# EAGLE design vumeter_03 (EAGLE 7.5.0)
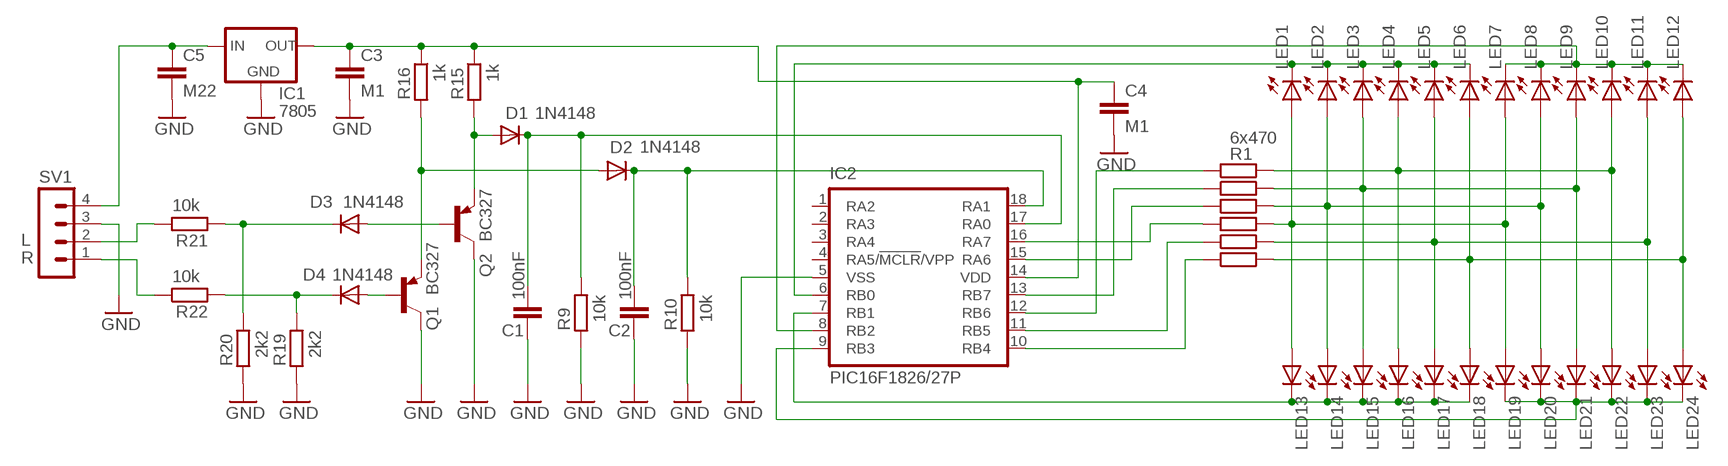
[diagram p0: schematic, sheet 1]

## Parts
C1  100nF  C-EU050-024X044  [C050-024X044]
C2  100nF  C-EU050-024X044  [C050-024X044]
C3  M1  C-EU050-024X044  [C050-024X044]
C4  M1  C-EU050-024X044  [C050-024X044]
C5  M22  C-EU050-024X044  [C050-024X044]
D1  1N4148  DIODE-D-7.5  [D-7.5]
D2  1N4148  DIODE-D-7.5  [D-7.5]
D3  1N4148  DIODE-D-7.5  [D-7.5]
D4  1N4148  DIODE-D-7.5  [D-7.5]
IC1  7805  78XXL  [78XXL]
IC2  PIC16F1826/27P  [DIL18]
LED1  LED5MM  [LED5MM]
LED2  LED5MM  [LED5MM]
LED3  LED5MM  [LED5MM]
LED4  LED5MM  [LED5MM]
LED5  LED5MM  [LED5MM]
LED6  LED5MM  [LED5MM]
LED7  LED5MM  [LED5MM]
LED8  LED5MM  [LED5MM]
LED9  LED5MM  [LED5MM]
LED10  LED5MM  [LED5MM]
LED11  LED5MM  [LED5MM]
LED12  LED5MM  [LED5MM]
LED13  LED5MM  [LED5MM]
LED14  LED5MM  [LED5MM]
LED15  LED5MM  [LED5MM]
LED16  LED5MM  [LED5MM]
LED17  LED5MM  [LED5MM]
LED18  LED5MM  [LED5MM]
LED19  LED5MM  [LED5MM]
LED20  LED5MM  [LED5MM]
LED21  LED5MM  [LED5MM]
LED22  LED5MM  [LED5MM]
LED23  LED5MM  [LED5MM]
LED24  LED5MM  [LED5MM]
Q1  BC327  [TO92-EBC]
Q2  BC327  [TO92-EBC]
R1  470  R-EU_0207/10  [0207/10]
R2  470  R-EU_0207/10  [0207/10]
R3  470  R-EU_0207/10  [0207/10]
R4  470  R-EU_0207/10  [0207/10]
R5  470  R-EU_0207/10  [0207/10]
R6  470  R-EU_0207/10  [0207/10]
R9  10k  R-EU_0207/10  [0207/10]
R10  10k  R-EU_0207/10  [0207/10]
R15  1k  R-EU_0207/10  [0207/10]
R16  1k  R-EU_0207/10  [0207/10]
R19  2k2  R-EU_0207/10  [0207/10]
R20  2k2  R-EU_0207/10  [0207/10]
R21  10k  R-EU_0207/10  [0207/10]
R22  10k  R-EU_0207/10  [0207/10]
SV1  MA04-1  [MA04-1]

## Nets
AN0: C1.1 D1.C IC2.17(RA0) R9.1
AN1: C2.1 D2.C IC2.18(RA1) R10.1
ANODY_L1: IC2.6(RB0) LED1.K(C) LED2.K(C) LED3.K(C) LED4.K(C) LED5.K(C) LED6.K(C)
ANODY_L2: IC2.8(RB2) LED7.K(C) LED8.K(C) LED9.K(C) LED10.K(C) LED11.K(C) LED12.K(C)
ANODY_R1: IC2.7(RB1) LED13.K(C) LED14.K(C) LED15.K(C) LED16.K(C) LED17.K(C) LED18.K(C)
ANODY_R2: IC2.9(RB3) LED19.K(C) LED20.K(C) LED21.K(C) LED22.K(C) LED23.K(C) LED24.K(C)
GND: C1.2 C2.2 C3.2 C4.2 C5.2 IC1.GND IC2.5(VSS) Q1.C Q2.C R9.2 R10.2 R19.2 R20.2 SV1.3
N$1: LED1.A LED7.A LED13.A LED19.A R4.2
N$2: LED2.A LED8.A LED14.A LED20.A R3.2
N$3: LED5.A LED11.A LED17.A LED23.A R5.2
N$4: LED4.A LED10.A LED16.A LED22.A R1.2
N$5: D4.A Q1.B
N$6: C5.1 IC1.IN SV1.4
N$7: D2.A Q1.E R16.2
N$8: LED6.A LED12.A LED18.A LED24.A R6.2
N$9: IC2.10(RB4) R6.1
N$10: IC2.11(RB5) R5.1
N$11: LED3.A LED9.A LED15.A LED21.A R2.2
N$12: IC2.16(RA7) R4.1
N$13: D1.A Q2.E R15.2
N$14: IC2.15(RA6) R3.1
N$15: IC2.13(RB7) R2.1
N$16: IC2.12(RB6) R1.1
N$17: D3.A Q2.B
N$18: R21.1 SV1.2
N$19: R22.1 SV1.1
N$20: C3.1 C4.1 IC1.OUT IC2.14(VDD) R15.1 R16.1
N$22: D3.C R20.1 R21.2
N$23: D4.C R19.1 R22.2
Unconnected: IC2.1(RA2) IC2.2(RA3) IC2.3(RA4) IC2.4(RA5/!MCLR!/VPP)

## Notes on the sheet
- 6x470
- L
- R

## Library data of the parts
C1-C5 = rcl:C-EU: CAPACITOR, European symbol
D1-D4 = diode:DIODE-: DIODE
IC1 = v-reg:78XXL: VOLTAGE REGULATOR
IC2 = microchip:PIC16*F1826/27: 18/20/28-Pin Flash Microcontrollers with nanoWatt XLP Technology Source: www.microchip.com PIC16F1827.pdf
LED1-LED24 = led:LED: LED
Q1 Q2 = transistor-pnp:BC327*: PNP Transistror
R1-R6 R9 R10 R15 R16 R19-R22 = rcl:R-EU_: RESISTOR, European symbol
SV1 = con-lstb:MA04-1: PIN HEADER

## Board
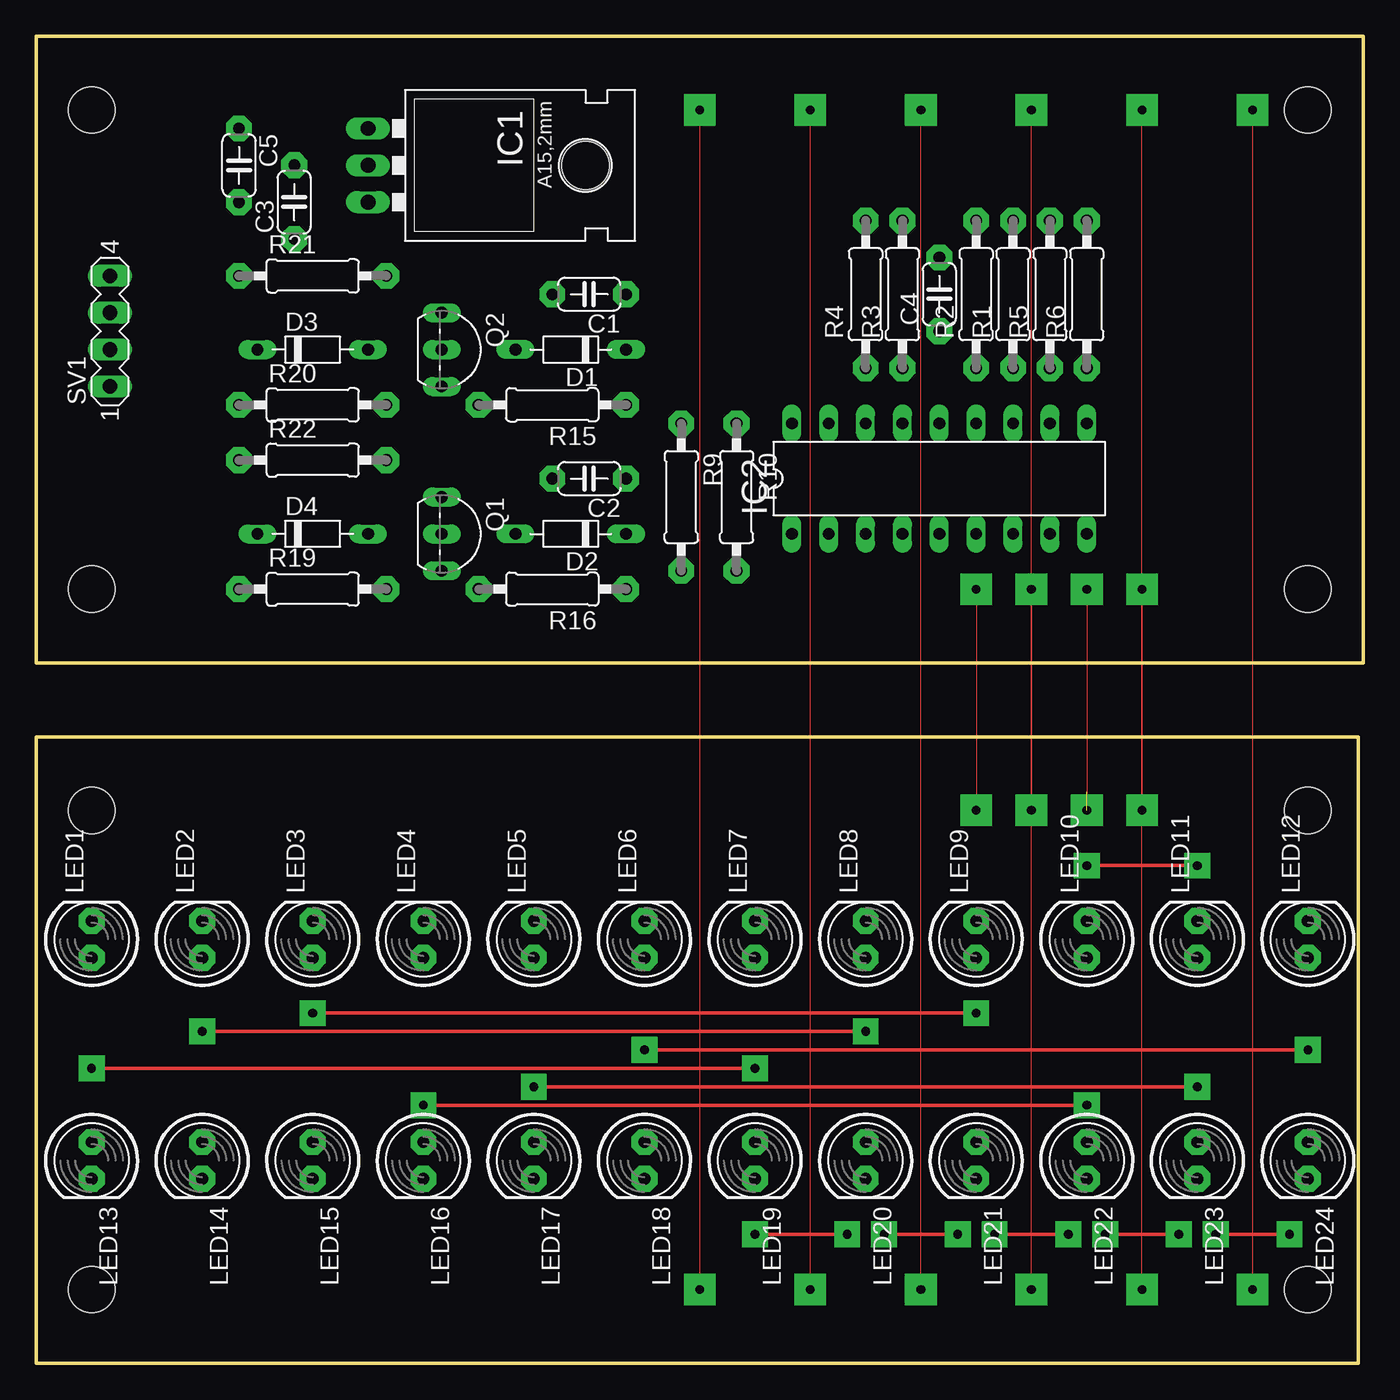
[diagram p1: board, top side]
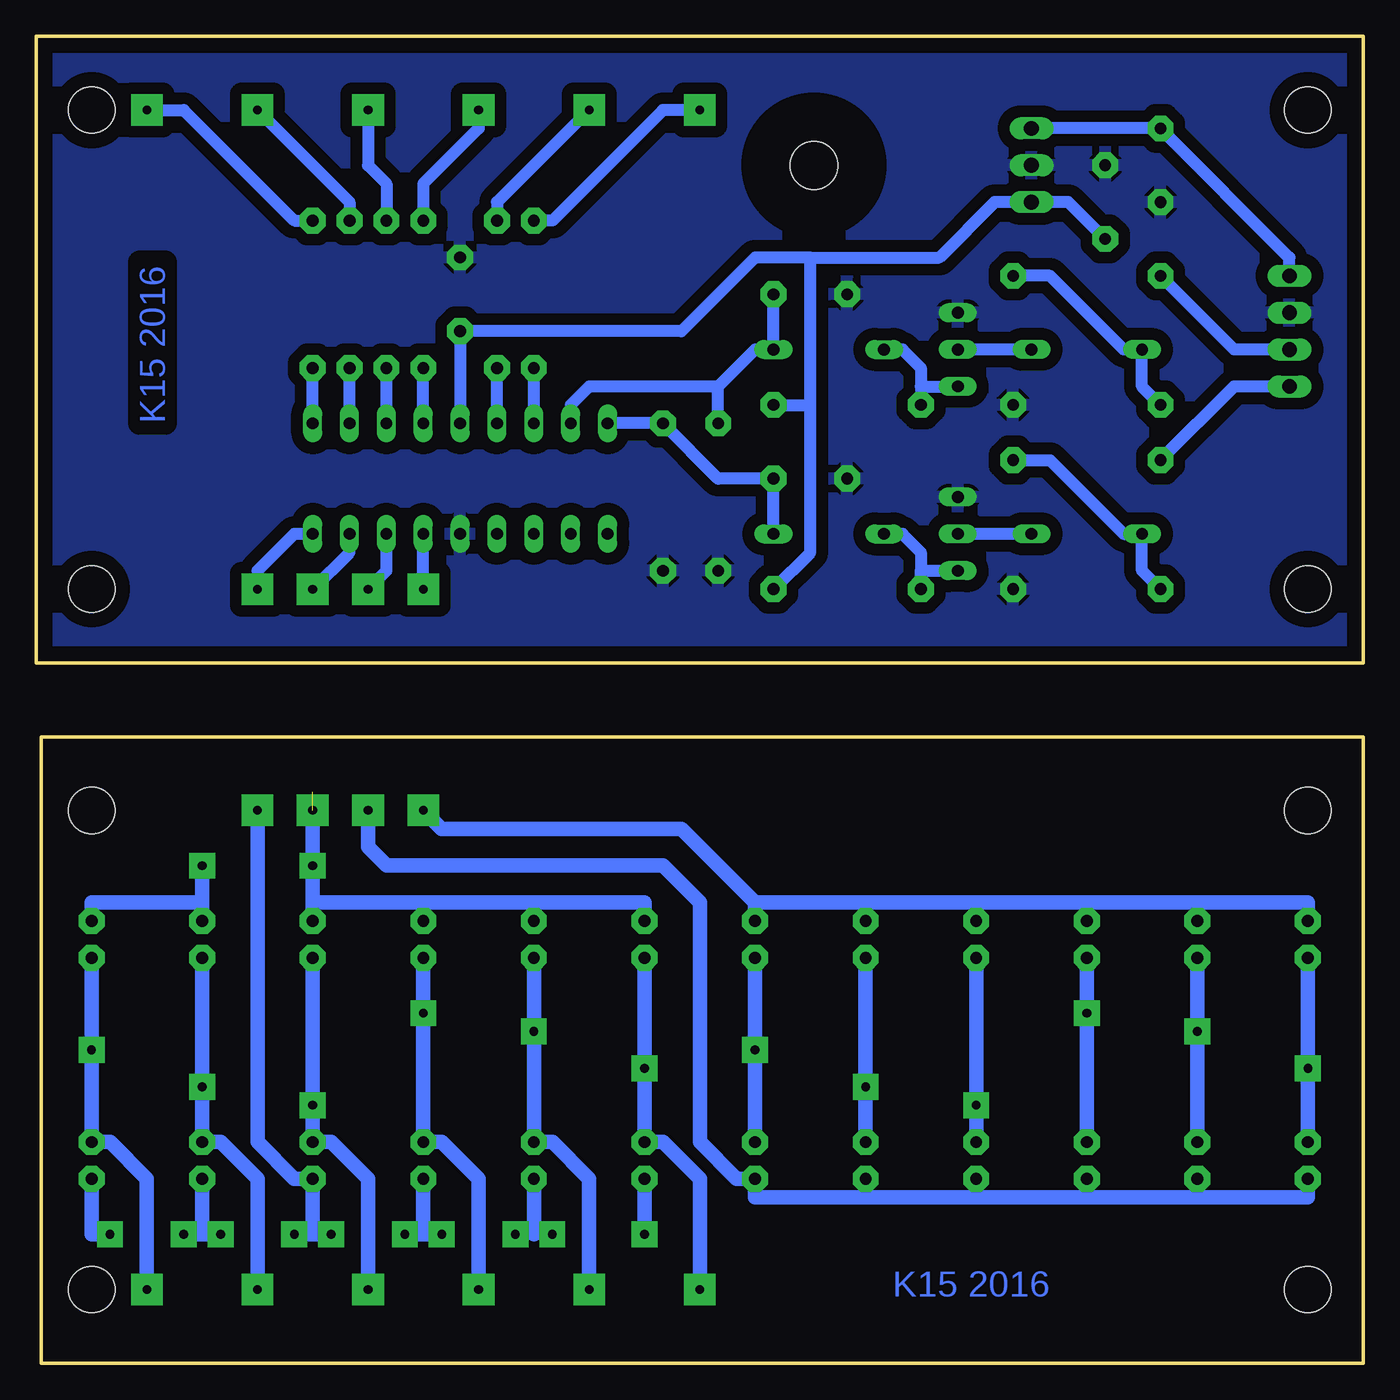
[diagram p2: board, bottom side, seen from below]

Size 91.44 x 91.44 mm. Coordinates in mm from the lower left corner, seen from the top.
Outline: 0,0 91.11,0 91.11,43.17 0,43.17 0,0
Outline: 0,48.26 91.44,48.26 91.44,91.44 0,91.44 0,48.26
Copper layers (1*16): Top 0.035mm / dielectric 1.5mm / Bottom 0.035mm
Design rules "default": minimum track width 10mil, minimum drill 24mil, track to track 8mil, track to pad 8mil, pad to pad 8mil, via to via 8mil, smd to smd 8mil, copper to edge 40mil, drill to drill 8mil, minimum pad ring 10mil, minimum via ring 8mil, stop-mask expansion 4mil, vias tented up to drill 0mil, thermal gap 10mil
Holes 3.2 mm at 3.81,38.1 87.63,5.08 87.63,53.34 3.81,53.34 87.63,38.1 3.81,5.08 87.63,86.36 3.81,86.36

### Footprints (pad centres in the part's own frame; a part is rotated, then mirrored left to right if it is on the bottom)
C050-024X044 = drill 0.813 pad 1.778 octagon: 1 -2.54,0; 2 2.54,0
D-7.5 = drill 0.813 long: A 3.81,0; C -3.81,0
78XXL = drill 1.016 long: GND 0,-3.81; IN -2.54,-3.81; OUT 2.54,-3.81 | hole 3.302: 0,11.176
DIL18 = drill 0.813 long: 1 -10.16,-3.81; 2 -7.62,-3.81; 3 -5.08,-3.81; 4 -2.54,-3.81; 5 0,-3.81; 6 2.54,-3.81; 7 5.08,-3.81; 8 7.62,-3.81; 9 10.16,-3.81; 10 10.16,3.81; 11 7.62,3.81; 12 5.08,3.81; 13 2.54,3.81; 14 0,3.81; 15 -2.54,3.81; 16 -5.08,3.81; 17 -7.62,3.81; 18 -10.16,3.81
LED5MM = drill 0.813 pad 1.778 octagon: A -1.27,0; K 1.27,0
TO92-EBC = drill 0.813 long: B 0,-1.27; C -2.54,-1.27; E 2.54,-1.27
0207/10 = drill 0.813 pad 1.778 octagon: 1 -5.08,0; 2 5.08,0
MA04-1 = drill 1.016 long: 1 -3.81,0; 2 -1.27,0; 3 1.27,0; 4 3.81,0

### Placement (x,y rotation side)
C1  38.1,73.66 180 top
C2  38.1,60.96 180 top
C3  17.78,80.01 90 top
C4  62.23,73.66 90 top
C5  13.97,82.55 270 top
D1  36.83,69.85 180 top
D2  36.83,57.15 180 top
D3  19.05,69.85 0 top
D4  19.05,57.15 0 top
IC1  26.67,82.55 270 top
IC2  62.23,60.96 0 top
LED1  3.81,29.21 90 top
LED2  11.43,29.21 90 top
LED3  19.05,29.21 90 top
LED4  26.67,29.21 90 top
LED5  34.29,29.21 90 top
LED6  41.91,29.21 90 top
LED7  49.53,29.21 90 top
LED8  57.15,29.21 90 top
LED9  64.77,29.21 90 top
LED10  72.39,29.21 90 top
LED11  80.01,29.21 90 top
LED12  87.63,29.21 90 top
LED13  3.81,13.97 270 top
LED14  11.43,13.97 270 top
LED15  19.05,13.97 270 top
LED16  26.67,13.97 270 top
LED17  34.29,13.97 270 top
LED18  41.91,13.97 270 top
LED19  49.53,13.97 270 top
LED20  57.15,13.97 270 top
LED21  64.77,13.97 270 top
LED22  72.39,13.97 270 top
LED23  80.01,13.97 270 top
LED24  87.63,13.97 270 top
Q1  29.21,57.15 270 top
Q2  29.21,69.85 270 top
R1  67.31,73.66 90 top
R2  64.77,73.66 90 top
R3  59.69,73.66 90 top
R4  57.15,73.66 90 top
R5  69.85,73.66 90 top
R6  72.39,73.66 90 top
R9  44.45,59.69 270 top
R10  48.26,59.69 270 top
R15  35.56,66.04 180 top
R16  35.56,53.34 180 top
R19  19.05,53.34 0 top
R20  19.05,66.04 0 top
R21  19.05,74.93 0 top
R22  19.05,62.23 0 top
SV1  5.08,71.12 90 top

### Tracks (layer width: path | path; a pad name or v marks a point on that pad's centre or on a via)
AN0
  Bottom 0.813: C1.1 D1.C 41.91,69.85 44.45,67.31 | IC2.17 54.61,66.04 53.34,67.31 44.45,67.31 | R9.1 44.45,67.31
AN1
  Bottom 0.813: D2.C C2.1 44.45,60.96 R10.1 IC2.18
ANODY_L1  (via drill 0.6 pad 2.18)
  Top 0: v64.77,53.34 v64.77,38.1
  Bottom 0.813: v64.77,53.34 IC2.6
  Bottom 1.016: 11.43,31.75 3.81,31.75 LED1.K | 11.43,31.75 19.05,31.75 | 19.05,31.75 26.67,31.75 | 26.67,31.75 34.29,31.75 | 34.29,31.75 41.91,31.75 | v64.77,38.1 63.5,36.83 46.99,36.83 41.91,31.75 | LED2.K 11.43,31.75 | LED3.K 19.05,31.75 | LED4.K 26.67,31.75 | LED5.K 34.29,31.75 | LED6.K 41.91,31.75
ANODY_L2  (via drill 0.6 pad 1.78, 0.6 pad 2.18)  (1 unrouted)
  Top 0: v72.39,53.34 v72.39,38.1
  Top 0.254: v80.01,34.29 v72.39,34.29
  Bottom 0.813: v72.39,53.34 69.85,55.88 IC2.8
  Bottom 1.016: v72.39,38.1 v72.39,34.29 72.39,31.75 | 80.01,31.75 87.63,31.75 LED12.K | 57.15,31.75 49.53,31.75 LED7.K | 57.15,31.75 64.77,31.75 | 64.77,31.75 72.39,31.75 | LED8.K 57.15,31.75 | LED9.K 64.77,31.75 | LED10.K 72.39,31.75 | LED11.K 80.01,31.75 | 80.01,31.75 v80.01,34.29
ANODY_R1  (via drill 0.6 pad 2.18)
  Top 0: v68.58,53.34 v68.58,38.1
  Bottom 0.813: v68.58,53.34 67.31,54.61 IC2.7
  Bottom 1.016: 11.43,11.43 3.81,11.43 LED13.K | 11.43,11.43 19.05,11.43 | 19.05,11.43 26.67,11.43 | 26.67,11.43 34.29,11.43 | 34.29,11.43 41.91,11.43 LED18.K 43.18,12.7 45.72,15.24 45.72,31.75 48.26,34.29 67.31,34.29 68.58,35.56 v68.58,38.1 | LED14.K 11.43,11.43 | LED15.K 19.05,11.43 | LED16.K 26.67,11.43 | LED17.K 34.29,11.43
ANODY_R2  (via drill 0.6 pad 1.78, 0.6 pad 2.18)
  Top 0: v76.2,53.34 v76.2,38.1
  Top 0.254: v49.53,8.89 v55.88,8.89 | v58.42,8.89 v63.5,8.89 | v66.04,8.89 v71.12,8.89 | v78.74,8.89 v73.66,8.89 | v81.28,8.89 v86.36,8.89
  Bottom 0.813: IC2.9 73.66,57.15 76.2,54.61 v76.2,53.34 | v55.88,8.89 57.15,8.89 v58.42,8.89
  Bottom 1.016: v76.2,38.1 76.2,15.24 73.66,12.7 LED22.K 72.39,8.89 | LED19.K v49.53,8.89 | LED20.K 57.15,8.89 | v63.5,8.89 64.77,8.89 | LED21.K 64.77,8.89 | 64.77,8.89 v66.04,8.89 | v71.12,8.89 72.39,8.89 | 80.01,8.89 v78.74,8.89 | v73.66,8.89 72.39,8.89 | LED23.K 80.01,8.89 | 80.01,8.89 v81.28,8.89 | v86.36,8.89 87.63,8.89 LED24.K
GND
  pour Bottom (isolate 0.813): -1.27,46.99 -1.27,92.71 92.71,92.71 92.71,46.99
N$1  (via drill 0.6 pad 1.78, 0.6 pad 2.18)
  Top 0: v45.72,5.08 v45.72,86.36
  Top 0.254: v3.81,20.32 v49.53,20.32
  Bottom 0.813: v45.72,86.36 48.26,86.36 55.88,78.74 R4.2
  Bottom 1.016: v45.72,5.08 45.72,12.7 48.26,15.24 LED19.A v49.53,20.32 LED7.A | LED13.A v3.81,20.32 LED1.A
N$2  (via drill 0.6 pad 1.78, 0.6 pad 2.18)
  Top 0: v53.34,5.08 v53.34,86.36
  Top 0.254: v11.43,22.86 v57.15,22.86
  Bottom 0.813: v53.34,86.36 59.69,80.01 R3.2
  Bottom 1.016: v53.34,5.08 53.34,12.7 55.88,15.24 LED20.A v57.15,22.86 LED8.A | LED2.A v11.43,22.86 LED14.A
N$3  (via drill 0.6 pad 1.78, 0.6 pad 2.18)
  Top 0: v76.2,5.08 v76.2,86.36
  Top 0.254: v34.29,19.05 v80.01,19.05
  Bottom 0.813: v76.2,86.36 69.85,80.01 R5.2
  Bottom 1.016: v76.2,5.08 76.2,12.7 78.74,15.24 LED23.A v80.01,19.05 LED11.A | LED5.A v34.29,19.05 LED17.A
N$4  (via drill 0.6 pad 1.78, 0.6 pad 2.18)
  Top 0: v68.58,5.08 v68.58,86.36
  Top 0.254: v26.67,17.78 v72.39,17.78
  Bottom 0.813: v68.58,86.36 68.58,82.55 67.31,81.28 R1.2
  Bottom 1.016: v68.58,5.08 68.58,12.7 71.12,15.24 LED22.A v72.39,17.78 LED10.A | LED4.A v26.67,17.78 LED16.A
N$5
  Bottom 0.813: D4.A Q1.B
N$6
  Bottom 0.813: SV1.4 5.08,76.2 C5.1 IC1.IN
N$7
  Bottom 0.813: R16.2 30.48,54.61 | D2.A 31.75,57.15 30.48,55.88 30.48,54.61 | 30.48,54.61 Q1.E
N$8  (via drill 0.6 pad 1.78, 0.6 pad 2.18)
  Top 0: v83.82,5.08 v83.82,86.36
  Top 0.254: v41.91,21.59 v87.63,21.59
  Bottom 0.813: v83.82,86.36 81.28,86.36 73.66,78.74 R6.2
  Bottom 1.016: LED6.A v41.91,21.59 LED18.A | LED12.A v87.63,21.59 LED24.A 86.36,15.24 83.82,12.7 v83.82,5.08
N$9
  Bottom 0.813: IC2.10 R6.1
N$10
  Bottom 0.813: IC2.11 R5.1
N$11  (via drill 0.6 pad 1.78, 0.6 pad 2.18)
  Top 0: v60.96,5.08 v60.96,86.36
  Top 0.254: v19.05,24.13 v64.77,24.13
  Bottom 0.813: v60.96,86.36 60.96,85.09 64.77,81.28 R2.2
  Bottom 1.016: v60.96,5.08 60.96,12.7 63.5,15.24 LED21.A v64.77,24.13 LED9.A | LED3.A v19.05,24.13 LED15.A
N$12
  Bottom 0.813: IC2.16 R4.1
N$13
  Bottom 0.813: D1.A 31.75,69.85 30.48,68.58 30.48,67.31 | 30.48,67.31 Q2.E | 30.48,67.31 R15.2
N$14
  Bottom 0.813: IC2.15 R3.1
N$15
  Bottom 0.813: IC2.13 R2.1
N$16
  Bottom 0.813: IC2.12 R1.1
N$17
  Bottom 0.813: D3.A Q2.B
N$18
  Bottom 0.813: SV1.2 8.89,69.85 R21.1
N$19
  Bottom 0.813: SV1.1 8.89,67.31 R22.1
N$20
  Bottom 0.813: 38.1,76.2 29.21,76.2 25.4,80.01 IC1.OUT 20.32,80.01 C3.1 | R16.1 38.1,55.88 38.1,66.04 | 38.1,66.04 38.1,76.2 | R15.1 38.1,66.04 | 38.1,76.2 41.91,76.2 46.99,71.12 C4.1 IC2.14
N$22
  Bottom 0.813: R20.1 15.24,67.31 D3.C 16.51,69.85 21.59,74.93 R21.2
N$23
  Bottom 0.813: R19.1 15.24,54.61 D4.C 16.51,57.15 21.59,62.23 R22.2

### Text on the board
Bottom: K15 2016 | K15 2016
